DATA_BLOCK "IMAC_STANDBY_RECORD"
TITLE = STANDBY_RECORD
AUTHOR : HottendU
FAMILY : IMAC
VERSION : 0.2


  STRUCT
   STANDBY_No001 : STRUCT
    System : WORD ;
    CmdOS : WORD ;
    MirrorCmdOS : WORD ;
    Test : WORD ;
    AlarmOS : WORD ;
    StatusOS : WORD ;
    SysStatusOS : WORD ;
    Status1 : WORD ;
    Status2 : WORD ;
    Status3 : BYTE ;
    InputEdges : BYTE ;
    AutoEdges : WORD ;
    DataTimeCODelay : STRUCT
     StartTime : DINT ;
     StartEdge : BOOL ;
    END_STRUCT ;
    DataTimeStartingA : STRUCT
     StartTime : DINT ;
     StartEdge : BOOL ;
    END_STRUCT ;
    DataTimeStartingB : STRUCT
     StartTime : DINT ;
     StartEdge : BOOL ;
    END_STRUCT ;
    DataTimeFaultA : STRUCT
     StartTime : DINT ;
     StartEdge : BOOL ;
    END_STRUCT ;
    DataTimeFaultB : STRUCT
     StartTime : DINT ;
     StartEdge : BOOL ;
    END_STRUCT ;
    PCONF : STRUCT 	//// PCONF STANDBY - Instance 001
     Modeswitches : STRUCT
      M0_Spare : BOOL ;	// Spare
      M1_Spare : BOOL ;	// Spare
      M2_Spare : BOOL ;	// Spare
      M3_Spare : BOOL ;	// Spare
      M4_Spare : BOOL ;	// Spare
      M5_Spare : BOOL ;	// Spare
      M6_Spare : BOOL ;	// Spare
      M7_Spare : BOOL ;	// Spare
      M8_Spare : BOOL ;	// Spare
      M9_Spare : BOOL ;	// Spare
      M10_Spare : BOOL ;	// Spare
      M11_Spare : BOOL ;	// Spare
      M12_Spare : BOOL ;	// Spare
      M13_Spare : BOOL ;	// Spare
      M14_Spare : BOOL ;	// Spare
      M15_Test : BOOL ;	// Testbit (1)
     END_STRUCT ;
     DlyTCODelay : TIME  := T#10S;	// Setpoint Action Fault delay
     DlyTStartingA : TIME  := T#3S;	// Setpoint Waiting Delay Slow->Fast
     DlyTStartingB : TIME  := T#3S;	// Setpoint Waiting Delay Fast->Slow
     DlyTFaultA : TIME  := T#2S;	// Setpoint feedback fault delay
     DlyTFaultB : TIME  := T#2S;	// Setpoint change direction
    END_STRUCT ;
   END_STRUCT ;
   STANDBY_No002 : STRUCT
    System : WORD ;
    CmdOS : WORD ;
    MirrorCmdOS : WORD ;
    Test : WORD ;
    AlarmOS : WORD ;
    StatusOS : WORD ;
    SysStatusOS : WORD ;
    Status1 : WORD ;
    Status2 : WORD ;
    Status3 : BYTE ;
    InputEdges : BYTE ;
    AutoEdges : WORD ;
    DataTimeCODelay : STRUCT
     StartTime : DINT ;
     StartEdge : BOOL ;
    END_STRUCT ;
    DataTimeStartingA : STRUCT
     StartTime : DINT ;
     StartEdge : BOOL ;
    END_STRUCT ;
    DataTimeStartingB : STRUCT
     StartTime : DINT ;
     StartEdge : BOOL ;
    END_STRUCT ;
    DataTimeFaultA : STRUCT
     StartTime : DINT ;
     StartEdge : BOOL ;
    END_STRUCT ;
    DataTimeFaultB : STRUCT
     StartTime : DINT ;
     StartEdge : BOOL ;
    END_STRUCT ;
    PCONF : STRUCT 	//// PCONF STANDBY - Instance 002
     Modeswitches : STRUCT
      M0_Spare : BOOL ;	// Spare
      M1_Spare : BOOL ;	// Spare
      M2_Spare : BOOL ;	// Spare
      M3_Spare : BOOL ;	// Spare
      M4_Spare : BOOL ;	// Spare
      M5_Spare : BOOL ;	// Spare
      M6_Spare : BOOL ;	// Spare
      M7_Spare : BOOL ;	// Spare
      M8_Spare : BOOL ;	// Spare
      M9_Spare : BOOL ;	// Spare
      M10_Spare : BOOL ;	// Spare
      M11_Spare : BOOL ;	// Spare
      M12_Spare : BOOL ;	// Spare
      M13_Spare : BOOL ;	// Spare
      M14_Spare : BOOL ;	// Spare
      M15_Test : BOOL ;	// Testbit (1)
     END_STRUCT ;
     DlyTCODelay : TIME ;	// Setpoint Action Fault delay
     DlyTStartingA : TIME ;	// Setpoint Waiting Delay Slow->Fast
     DlyTStartingB : TIME ;	// Setpoint Waiting Delay Fast->Slow
     DlyTFaultA : TIME ;	// Setpoint feedback fault delay
     DlyTFaultB : TIME ;	// Setpoint change direction
    END_STRUCT ;
   END_STRUCT ;
   STANDBY_No003 : STRUCT
    System : WORD ;
    CmdOS : WORD ;
    MirrorCmdOS : WORD ;
    Test : WORD ;
    AlarmOS : WORD ;
    StatusOS : WORD ;
    SysStatusOS : WORD ;
    Status1 : WORD ;
    Status2 : WORD ;
    Status3 : BYTE ;
    InputEdges : BYTE ;
    AutoEdges : WORD ;
    DataTimeCODelay : STRUCT
     StartTime : DINT ;
     StartEdge : BOOL ;
    END_STRUCT ;
    DataTimeStartingA : STRUCT
     StartTime : DINT ;
     StartEdge : BOOL ;
    END_STRUCT ;
    DataTimeStartingB : STRUCT
     StartTime : DINT ;
     StartEdge : BOOL ;
    END_STRUCT ;
    DataTimeFaultA : STRUCT
     StartTime : DINT ;
     StartEdge : BOOL ;
    END_STRUCT ;
    DataTimeFaultB : STRUCT
     StartTime : DINT ;
     StartEdge : BOOL ;
    END_STRUCT ;
    PCONF : STRUCT 	//// PCONF STANDBY - Instance 003
     Modeswitches : STRUCT
      M0_Spare : BOOL ;	// Spare
      M1_Spare : BOOL ;	// Spare
      M2_Spare : BOOL ;	// Spare
      M3_Spare : BOOL ;	// Spare
      M4_Spare : BOOL ;	// Spare
      M5_Spare : BOOL ;	// Spare
      M6_Spare : BOOL ;	// Spare
      M7_Spare : BOOL ;	// Spare
      M8_Spare : BOOL ;	// Spare
      M9_Spare : BOOL ;	// Spare
      M10_Spare : BOOL ;	// Spare
      M11_Spare : BOOL ;	// Spare
      M12_Spare : BOOL ;	// Spare
      M13_Spare : BOOL ;	// Spare
      M14_Spare : BOOL ;	// Spare
      M15_Test : BOOL ;	// Testbit (1)
     END_STRUCT ;
     DlyTCODelay : TIME ;	// Setpoint Action Fault delay
     DlyTStartingA : TIME ;	// Setpoint Waiting Delay Slow->Fast
     DlyTStartingB : TIME ;	// Setpoint Waiting Delay Fast->Slow
     DlyTFaultA : TIME ;	// Setpoint feedback fault delay
     DlyTFaultB : TIME ;	// Setpoint change direction
    END_STRUCT ;
   END_STRUCT ;
   STANDBY_No004 : STRUCT
    System : WORD ;
    CmdOS : WORD ;
    MirrorCmdOS : WORD ;
    Test : WORD ;
    AlarmOS : WORD ;
    StatusOS : WORD ;
    SysStatusOS : WORD ;
    Status1 : WORD ;
    Status2 : WORD ;
    Status3 : BYTE ;
    InputEdges : BYTE ;
    AutoEdges : WORD ;
    DataTimeCODelay : STRUCT
     StartTime : DINT ;
     StartEdge : BOOL ;
    END_STRUCT ;
    DataTimeStartingA : STRUCT
     StartTime : DINT ;
     StartEdge : BOOL ;
    END_STRUCT ;
    DataTimeStartingB : STRUCT
     StartTime : DINT ;
     StartEdge : BOOL ;
    END_STRUCT ;
    DataTimeFaultA : STRUCT
     StartTime : DINT ;
     StartEdge : BOOL ;
    END_STRUCT ;
    DataTimeFaultB : STRUCT
     StartTime : DINT ;
     StartEdge : BOOL ;
    END_STRUCT ;
    PCONF : STRUCT 	//// PCONF STANDBY - Instance 004
     Modeswitches : STRUCT
      M0_Spare : BOOL ;	// Spare
      M1_Spare : BOOL ;	// Spare
      M2_Spare : BOOL ;	// Spare
      M3_Spare : BOOL ;	// Spare
      M4_Spare : BOOL ;	// Spare
      M5_Spare : BOOL ;	// Spare
      M6_Spare : BOOL ;	// Spare
      M7_Spare : BOOL ;	// Spare
      M8_Spare : BOOL ;	// Spare
      M9_Spare : BOOL ;	// Spare
      M10_Spare : BOOL ;	// Spare
      M11_Spare : BOOL ;	// Spare
      M12_Spare : BOOL ;	// Spare
      M13_Spare : BOOL ;	// Spare
      M14_Spare : BOOL ;	// Spare
      M15_Test : BOOL ;	// Testbit (1)
     END_STRUCT ;
     DlyTCODelay : TIME ;	// Setpoint Action Fault delay
     DlyTStartingA : TIME ;	// Setpoint Waiting Delay Slow->Fast
     DlyTStartingB : TIME ;	// Setpoint Waiting Delay Fast->Slow
     DlyTFaultA : TIME ;	// Setpoint feedback fault delay
     DlyTFaultB : TIME ;	// Setpoint change direction
    END_STRUCT ;
   END_STRUCT ;
   STANDBY_No005 : STRUCT
    System : WORD ;
    CmdOS : WORD ;
    MirrorCmdOS : WORD ;
    Test : WORD ;
    AlarmOS : WORD ;
    StatusOS : WORD ;
    SysStatusOS : WORD ;
    Status1 : WORD ;
    Status2 : WORD ;
    Status3 : BYTE ;
    InputEdges : BYTE ;
    AutoEdges : WORD ;
    DataTimeCODelay : STRUCT
     StartTime : DINT ;
     StartEdge : BOOL ;
    END_STRUCT ;
    DataTimeStartingA : STRUCT
     StartTime : DINT ;
     StartEdge : BOOL ;
    END_STRUCT ;
    DataTimeStartingB : STRUCT
     StartTime : DINT ;
     StartEdge : BOOL ;
    END_STRUCT ;
    DataTimeFaultA : STRUCT
     StartTime : DINT ;
     StartEdge : BOOL ;
    END_STRUCT ;
    DataTimeFaultB : STRUCT
     StartTime : DINT ;
     StartEdge : BOOL ;
    END_STRUCT ;
    PCONF : STRUCT 	//// PCONF STANDBY - Instance 005
     Modeswitches : STRUCT
      M0_Spare : BOOL ;	// Spare
      M1_Spare : BOOL ;	// Spare
      M2_Spare : BOOL ;	// Spare
      M3_Spare : BOOL ;	// Spare
      M4_Spare : BOOL ;	// Spare
      M5_Spare : BOOL ;	// Spare
      M6_Spare : BOOL ;	// Spare
      M7_Spare : BOOL ;	// Spare
      M8_Spare : BOOL ;	// Spare
      M9_Spare : BOOL ;	// Spare
      M10_Spare : BOOL ;	// Spare
      M11_Spare : BOOL ;	// Spare
      M12_Spare : BOOL ;	// Spare
      M13_Spare : BOOL ;	// Spare
      M14_Spare : BOOL ;	// Spare
      M15_Test : BOOL ;	// Testbit (1)
     END_STRUCT ;
     DlyTCODelay : TIME ;	// Setpoint Action Fault delay
     DlyTStartingA : TIME ;	// Setpoint Waiting Delay Slow->Fast
     DlyTStartingB : TIME ;	// Setpoint Waiting Delay Fast->Slow
     DlyTFaultA : TIME ;	// Setpoint feedback fault delay
     DlyTFaultB : TIME ;	// Setpoint change direction
    END_STRUCT ;
   END_STRUCT ;
   STANDBY_No006 : STRUCT
    System : WORD ;
    CmdOS : WORD ;
    MirrorCmdOS : WORD ;
    Test : WORD ;
    AlarmOS : WORD ;
    StatusOS : WORD ;
    SysStatusOS : WORD ;
    Status1 : WORD ;
    Status2 : WORD ;
    Status3 : BYTE ;
    InputEdges : BYTE ;
    AutoEdges : WORD ;
    DataTimeCODelay : STRUCT
     StartTime : DINT ;
     StartEdge : BOOL ;
    END_STRUCT ;
    DataTimeStartingA : STRUCT
     StartTime : DINT ;
     StartEdge : BOOL ;
    END_STRUCT ;
    DataTimeStartingB : STRUCT
     StartTime : DINT ;
     StartEdge : BOOL ;
    END_STRUCT ;
    DataTimeFaultA : STRUCT
     StartTime : DINT ;
     StartEdge : BOOL ;
    END_STRUCT ;
    DataTimeFaultB : STRUCT
     StartTime : DINT ;
     StartEdge : BOOL ;
    END_STRUCT ;
    PCONF : STRUCT 	//// PCONF STANDBY - Instance 006
     Modeswitches : STRUCT
      M0_Spare : BOOL ;	// Spare
      M1_Spare : BOOL ;	// Spare
      M2_Spare : BOOL ;	// Spare
      M3_Spare : BOOL ;	// Spare
      M4_Spare : BOOL ;	// Spare
      M5_Spare : BOOL ;	// Spare
      M6_Spare : BOOL ;	// Spare
      M7_Spare : BOOL ;	// Spare
      M8_Spare : BOOL ;	// Spare
      M9_Spare : BOOL ;	// Spare
      M10_Spare : BOOL ;	// Spare
      M11_Spare : BOOL ;	// Spare
      M12_Spare : BOOL ;	// Spare
      M13_Spare : BOOL ;	// Spare
      M14_Spare : BOOL ;	// Spare
      M15_Test : BOOL ;	// Testbit (1)
     END_STRUCT ;
     DlyTCODelay : TIME ;	// Setpoint Action Fault delay
     DlyTStartingA : TIME ;	// Setpoint Waiting Delay Slow->Fast
     DlyTStartingB : TIME ;	// Setpoint Waiting Delay Fast->Slow
     DlyTFaultA : TIME ;	// Setpoint feedback fault delay
     DlyTFaultB : TIME ;	// Setpoint change direction
    END_STRUCT ;
   END_STRUCT ;
   STANDBY_No007 : STRUCT
    System : WORD ;
    CmdOS : WORD ;
    MirrorCmdOS : WORD ;
    Test : WORD ;
    AlarmOS : WORD ;
    StatusOS : WORD ;
    SysStatusOS : WORD ;
    Status1 : WORD ;
    Status2 : WORD ;
    Status3 : BYTE ;
    InputEdges : BYTE ;
    AutoEdges : WORD ;
    DataTimeCODelay : STRUCT
     StartTime : DINT ;
     StartEdge : BOOL ;
    END_STRUCT ;
    DataTimeStartingA : STRUCT
     StartTime : DINT ;
     StartEdge : BOOL ;
    END_STRUCT ;
    DataTimeStartingB : STRUCT
     StartTime : DINT ;
     StartEdge : BOOL ;
    END_STRUCT ;
    DataTimeFaultA : STRUCT
     StartTime : DINT ;
     StartEdge : BOOL ;
    END_STRUCT ;
    DataTimeFaultB : STRUCT
     StartTime : DINT ;
     StartEdge : BOOL ;
    END_STRUCT ;
    PCONF : STRUCT 	//// PCONF STANDBY - Instance 007
     Modeswitches : STRUCT
      M0_Spare : BOOL ;	// Spare
      M1_Spare : BOOL ;	// Spare
      M2_Spare : BOOL ;	// Spare
      M3_Spare : BOOL ;	// Spare
      M4_Spare : BOOL ;	// Spare
      M5_Spare : BOOL ;	// Spare
      M6_Spare : BOOL ;	// Spare
      M7_Spare : BOOL ;	// Spare
      M8_Spare : BOOL ;	// Spare
      M9_Spare : BOOL ;	// Spare
      M10_Spare : BOOL ;	// Spare
      M11_Spare : BOOL ;	// Spare
      M12_Spare : BOOL ;	// Spare
      M13_Spare : BOOL ;	// Spare
      M14_Spare : BOOL ;	// Spare
      M15_Test : BOOL ;	// Testbit (1)
     END_STRUCT ;
     DlyTCODelay : TIME ;	// Setpoint Action Fault delay
     DlyTStartingA : TIME ;	// Setpoint Waiting Delay Slow->Fast
     DlyTStartingB : TIME ;	// Setpoint Waiting Delay Fast->Slow
     DlyTFaultA : TIME ;	// Setpoint feedback fault delay
     DlyTFaultB : TIME ;	// Setpoint change direction
    END_STRUCT ;
   END_STRUCT ;
   STANDBY_No008 : STRUCT
    System : WORD ;
    CmdOS : WORD ;
    MirrorCmdOS : WORD ;
    Test : WORD ;
    AlarmOS : WORD ;
    StatusOS : WORD ;
    SysStatusOS : WORD ;
    Status1 : WORD ;
    Status2 : WORD ;
    Status3 : BYTE ;
    InputEdges : BYTE ;
    AutoEdges : WORD ;
    DataTimeCODelay : STRUCT
     StartTime : DINT ;
     StartEdge : BOOL ;
    END_STRUCT ;
    DataTimeStartingA : STRUCT
     StartTime : DINT ;
     StartEdge : BOOL ;
    END_STRUCT ;
    DataTimeStartingB : STRUCT
     StartTime : DINT ;
     StartEdge : BOOL ;
    END_STRUCT ;
    DataTimeFaultA : STRUCT
     StartTime : DINT ;
     StartEdge : BOOL ;
    END_STRUCT ;
    DataTimeFaultB : STRUCT
     StartTime : DINT ;
     StartEdge : BOOL ;
    END_STRUCT ;
    PCONF : STRUCT 	//// PCONF STANDBY - Instance 008
     Modeswitches : STRUCT
      M0_Spare : BOOL ;	// Spare
      M1_Spare : BOOL ;	// Spare
      M2_Spare : BOOL ;	// Spare
      M3_Spare : BOOL ;	// Spare
      M4_Spare : BOOL ;	// Spare
      M5_Spare : BOOL ;	// Spare
      M6_Spare : BOOL ;	// Spare
      M7_Spare : BOOL ;	// Spare
      M8_Spare : BOOL ;	// Spare
      M9_Spare : BOOL ;	// Spare
      M10_Spare : BOOL ;	// Spare
      M11_Spare : BOOL ;	// Spare
      M12_Spare : BOOL ;	// Spare
      M13_Spare : BOOL ;	// Spare
      M14_Spare : BOOL ;	// Spare
      M15_Test : BOOL ;	// Testbit (1)
     END_STRUCT ;
     DlyTCODelay : TIME ;	// Setpoint Action Fault delay
     DlyTStartingA : TIME ;	// Setpoint Waiting Delay Slow->Fast
     DlyTStartingB : TIME ;	// Setpoint Waiting Delay Fast->Slow
     DlyTFaultA : TIME ;	// Setpoint feedback fault delay
     DlyTFaultB : TIME ;	// Setpoint change direction
    END_STRUCT ;
   END_STRUCT ;
   STANDBY_No009 : STRUCT
    System : WORD ;
    CmdOS : WORD ;
    MirrorCmdOS : WORD ;
    Test : WORD ;
    AlarmOS : WORD ;
    StatusOS : WORD ;
    SysStatusOS : WORD ;
    Status1 : WORD ;
    Status2 : WORD ;
    Status3 : BYTE ;
    InputEdges : BYTE ;
    AutoEdges : WORD ;
    DataTimeCODelay : STRUCT
     StartTime : DINT ;
     StartEdge : BOOL ;
    END_STRUCT ;
    DataTimeStartingA : STRUCT
     StartTime : DINT ;
     StartEdge : BOOL ;
    END_STRUCT ;
    DataTimeStartingB : STRUCT
     StartTime : DINT ;
     StartEdge : BOOL ;
    END_STRUCT ;
    DataTimeFaultA : STRUCT
     StartTime : DINT ;
     StartEdge : BOOL ;
    END_STRUCT ;
    DataTimeFaultB : STRUCT
     StartTime : DINT ;
     StartEdge : BOOL ;
    END_STRUCT ;
    PCONF : STRUCT 	//// PCONF STANDBY - Instance 009
     Modeswitches : STRUCT
      M0_Spare : BOOL ;	// Spare
      M1_Spare : BOOL ;	// Spare
      M2_Spare : BOOL ;	// Spare
      M3_Spare : BOOL ;	// Spare
      M4_Spare : BOOL ;	// Spare
      M5_Spare : BOOL ;	// Spare
      M6_Spare : BOOL ;	// Spare
      M7_Spare : BOOL ;	// Spare
      M8_Spare : BOOL ;	// Spare
      M9_Spare : BOOL ;	// Spare
      M10_Spare : BOOL ;	// Spare
      M11_Spare : BOOL ;	// Spare
      M12_Spare : BOOL ;	// Spare
      M13_Spare : BOOL ;	// Spare
      M14_Spare : BOOL ;	// Spare
      M15_Test : BOOL ;	// Testbit (1)
     END_STRUCT ;
     DlyTCODelay : TIME ;	// Setpoint Action Fault delay
     DlyTStartingA : TIME ;	// Setpoint Waiting Delay Slow->Fast
     DlyTStartingB : TIME ;	// Setpoint Waiting Delay Fast->Slow
     DlyTFaultA : TIME ;	// Setpoint feedback fault delay
     DlyTFaultB : TIME ;	// Setpoint change direction
    END_STRUCT ;
   END_STRUCT ;
   STANDBY_No010 : STRUCT
    System : WORD ;
    CmdOS : WORD ;
    MirrorCmdOS : WORD ;
    Test : WORD ;
    AlarmOS : WORD ;
    StatusOS : WORD ;
    SysStatusOS : WORD ;
    Status1 : WORD ;
    Status2 : WORD ;
    Status3 : BYTE ;
    InputEdges : BYTE ;
    AutoEdges : WORD ;
    DataTimeCODelay : STRUCT
     StartTime : DINT ;
     StartEdge : BOOL ;
    END_STRUCT ;
    DataTimeStartingA : STRUCT
     StartTime : DINT ;
     StartEdge : BOOL ;
    END_STRUCT ;
    DataTimeStartingB : STRUCT
     StartTime : DINT ;
     StartEdge : BOOL ;
    END_STRUCT ;
    DataTimeFaultA : STRUCT
     StartTime : DINT ;
     StartEdge : BOOL ;
    END_STRUCT ;
    DataTimeFaultB : STRUCT
     StartTime : DINT ;
     StartEdge : BOOL ;
    END_STRUCT ;
    PCONF : STRUCT 	//// PCONF STANDBY - Instance 010
     Modeswitches : STRUCT
      M0_Spare : BOOL ;	// Spare
      M1_Spare : BOOL ;	// Spare
      M2_Spare : BOOL ;	// Spare
      M3_Spare : BOOL ;	// Spare
      M4_Spare : BOOL ;	// Spare
      M5_Spare : BOOL ;	// Spare
      M6_Spare : BOOL ;	// Spare
      M7_Spare : BOOL ;	// Spare
      M8_Spare : BOOL ;	// Spare
      M9_Spare : BOOL ;	// Spare
      M10_Spare : BOOL ;	// Spare
      M11_Spare : BOOL ;	// Spare
      M12_Spare : BOOL ;	// Spare
      M13_Spare : BOOL ;	// Spare
      M14_Spare : BOOL ;	// Spare
      M15_Test : BOOL ;	// Testbit (1)
     END_STRUCT ;
     DlyTCODelay : TIME ;	// Setpoint Action Fault delay
     DlyTStartingA : TIME ;	// Setpoint Waiting Delay Slow->Fast
     DlyTStartingB : TIME ;	// Setpoint Waiting Delay Fast->Slow
     DlyTFaultA : TIME ;	// Setpoint feedback fault delay
     DlyTFaultB : TIME ;	// Setpoint change direction
    END_STRUCT ;
   END_STRUCT ;
  END_STRUCT ;
BEGIN
   STANDBY_No001.System := W#16#0;
   STANDBY_No001.CmdOS := W#16#0;
   STANDBY_No001.MirrorCmdOS := W#16#0;
   STANDBY_No001.Test := W#16#0;
   STANDBY_No001.AlarmOS := W#16#0;
   STANDBY_No001.StatusOS := W#16#0;
   STANDBY_No001.SysStatusOS := W#16#0;
   STANDBY_No001.Status1 := W#16#0;
   STANDBY_No001.Status2 := W#16#0;
   STANDBY_No001.Status3 := B#16#0;
   STANDBY_No001.InputEdges := B#16#0;
   STANDBY_No001.AutoEdges := W#16#0;
   STANDBY_No001.DataTimeCODelay.StartTime := L#0;
   STANDBY_No001.DataTimeCODelay.StartEdge := FALSE;
   STANDBY_No001.DataTimeStartingA.StartTime := L#0;
   STANDBY_No001.DataTimeStartingA.StartEdge := FALSE;
   STANDBY_No001.DataTimeStartingB.StartTime := L#0;
   STANDBY_No001.DataTimeStartingB.StartEdge := FALSE;
   STANDBY_No001.DataTimeFaultA.StartTime := L#0;
   STANDBY_No001.DataTimeFaultA.StartEdge := FALSE;
   STANDBY_No001.DataTimeFaultB.StartTime := L#0;
   STANDBY_No001.DataTimeFaultB.StartEdge := FALSE;
   STANDBY_No001.PCONF.Modeswitches.M0_Spare := FALSE;
   STANDBY_No001.PCONF.Modeswitches.M1_Spare := FALSE;
   STANDBY_No001.PCONF.Modeswitches.M2_Spare := FALSE;
   STANDBY_No001.PCONF.Modeswitches.M3_Spare := FALSE;
   STANDBY_No001.PCONF.Modeswitches.M4_Spare := FALSE;
   STANDBY_No001.PCONF.Modeswitches.M5_Spare := FALSE;
   STANDBY_No001.PCONF.Modeswitches.M6_Spare := FALSE;
   STANDBY_No001.PCONF.Modeswitches.M7_Spare := FALSE;
   STANDBY_No001.PCONF.Modeswitches.M8_Spare := FALSE;
   STANDBY_No001.PCONF.Modeswitches.M9_Spare := FALSE;
   STANDBY_No001.PCONF.Modeswitches.M10_Spare := FALSE;
   STANDBY_No001.PCONF.Modeswitches.M11_Spare := FALSE;
   STANDBY_No001.PCONF.Modeswitches.M12_Spare := FALSE;
   STANDBY_No001.PCONF.Modeswitches.M13_Spare := FALSE;
   STANDBY_No001.PCONF.Modeswitches.M14_Spare := FALSE;
   STANDBY_No001.PCONF.Modeswitches.M15_Test := FALSE;
   STANDBY_No001.PCONF.DlyTCODelay := T#10S;
   STANDBY_No001.PCONF.DlyTStartingA := T#3S;
   STANDBY_No001.PCONF.DlyTStartingB := T#3S;
   STANDBY_No001.PCONF.DlyTFaultA := T#2S;
   STANDBY_No001.PCONF.DlyTFaultB := T#2S;
   STANDBY_No002.System := W#16#0;
   STANDBY_No002.CmdOS := W#16#0;
   STANDBY_No002.MirrorCmdOS := W#16#0;
   STANDBY_No002.Test := W#16#0;
   STANDBY_No002.AlarmOS := W#16#0;
   STANDBY_No002.StatusOS := W#16#0;
   STANDBY_No002.SysStatusOS := W#16#0;
   STANDBY_No002.Status1 := W#16#0;
   STANDBY_No002.Status2 := W#16#0;
   STANDBY_No002.Status3 := B#16#0;
   STANDBY_No002.InputEdges := B#16#0;
   STANDBY_No002.AutoEdges := W#16#0;
   STANDBY_No002.DataTimeCODelay.StartTime := L#0;
   STANDBY_No002.DataTimeCODelay.StartEdge := FALSE;
   STANDBY_No002.DataTimeStartingA.StartTime := L#0;
   STANDBY_No002.DataTimeStartingA.StartEdge := FALSE;
   STANDBY_No002.DataTimeStartingB.StartTime := L#0;
   STANDBY_No002.DataTimeStartingB.StartEdge := FALSE;
   STANDBY_No002.DataTimeFaultA.StartTime := L#0;
   STANDBY_No002.DataTimeFaultA.StartEdge := FALSE;
   STANDBY_No002.DataTimeFaultB.StartTime := L#0;
   STANDBY_No002.DataTimeFaultB.StartEdge := FALSE;
   STANDBY_No002.PCONF.Modeswitches.M0_Spare := FALSE;
   STANDBY_No002.PCONF.Modeswitches.M1_Spare := FALSE;
   STANDBY_No002.PCONF.Modeswitches.M2_Spare := FALSE;
   STANDBY_No002.PCONF.Modeswitches.M3_Spare := FALSE;
   STANDBY_No002.PCONF.Modeswitches.M4_Spare := FALSE;
   STANDBY_No002.PCONF.Modeswitches.M5_Spare := FALSE;
   STANDBY_No002.PCONF.Modeswitches.M6_Spare := FALSE;
   STANDBY_No002.PCONF.Modeswitches.M7_Spare := FALSE;
   STANDBY_No002.PCONF.Modeswitches.M8_Spare := FALSE;
   STANDBY_No002.PCONF.Modeswitches.M9_Spare := FALSE;
   STANDBY_No002.PCONF.Modeswitches.M10_Spare := FALSE;
   STANDBY_No002.PCONF.Modeswitches.M11_Spare := FALSE;
   STANDBY_No002.PCONF.Modeswitches.M12_Spare := FALSE;
   STANDBY_No002.PCONF.Modeswitches.M13_Spare := FALSE;
   STANDBY_No002.PCONF.Modeswitches.M14_Spare := FALSE;
   STANDBY_No002.PCONF.Modeswitches.M15_Test := FALSE;
   STANDBY_No002.PCONF.DlyTCODelay := T#0MS;
   STANDBY_No002.PCONF.DlyTStartingA := T#0MS;
   STANDBY_No002.PCONF.DlyTStartingB := T#0MS;
   STANDBY_No002.PCONF.DlyTFaultA := T#0MS;
   STANDBY_No002.PCONF.DlyTFaultB := T#0MS;
   STANDBY_No003.System := W#16#0;
   STANDBY_No003.CmdOS := W#16#0;
   STANDBY_No003.MirrorCmdOS := W#16#0;
   STANDBY_No003.Test := W#16#0;
   STANDBY_No003.AlarmOS := W#16#0;
   STANDBY_No003.StatusOS := W#16#0;
   STANDBY_No003.SysStatusOS := W#16#0;
   STANDBY_No003.Status1 := W#16#0;
   STANDBY_No003.Status2 := W#16#0;
   STANDBY_No003.Status3 := B#16#0;
   STANDBY_No003.InputEdges := B#16#0;
   STANDBY_No003.AutoEdges := W#16#0;
   STANDBY_No003.DataTimeCODelay.StartTime := L#0;
   STANDBY_No003.DataTimeCODelay.StartEdge := FALSE;
   STANDBY_No003.DataTimeStartingA.StartTime := L#0;
   STANDBY_No003.DataTimeStartingA.StartEdge := FALSE;
   STANDBY_No003.DataTimeStartingB.StartTime := L#0;
   STANDBY_No003.DataTimeStartingB.StartEdge := FALSE;
   STANDBY_No003.DataTimeFaultA.StartTime := L#0;
   STANDBY_No003.DataTimeFaultA.StartEdge := FALSE;
   STANDBY_No003.DataTimeFaultB.StartTime := L#0;
   STANDBY_No003.DataTimeFaultB.StartEdge := FALSE;
   STANDBY_No003.PCONF.Modeswitches.M0_Spare := FALSE;
   STANDBY_No003.PCONF.Modeswitches.M1_Spare := FALSE;
   STANDBY_No003.PCONF.Modeswitches.M2_Spare := FALSE;
   STANDBY_No003.PCONF.Modeswitches.M3_Spare := FALSE;
   STANDBY_No003.PCONF.Modeswitches.M4_Spare := FALSE;
   STANDBY_No003.PCONF.Modeswitches.M5_Spare := FALSE;
   STANDBY_No003.PCONF.Modeswitches.M6_Spare := FALSE;
   STANDBY_No003.PCONF.Modeswitches.M7_Spare := FALSE;
   STANDBY_No003.PCONF.Modeswitches.M8_Spare := FALSE;
   STANDBY_No003.PCONF.Modeswitches.M9_Spare := FALSE;
   STANDBY_No003.PCONF.Modeswitches.M10_Spare := FALSE;
   STANDBY_No003.PCONF.Modeswitches.M11_Spare := FALSE;
   STANDBY_No003.PCONF.Modeswitches.M12_Spare := FALSE;
   STANDBY_No003.PCONF.Modeswitches.M13_Spare := FALSE;
   STANDBY_No003.PCONF.Modeswitches.M14_Spare := FALSE;
   STANDBY_No003.PCONF.Modeswitches.M15_Test := FALSE;
   STANDBY_No003.PCONF.DlyTCODelay := T#0MS;
   STANDBY_No003.PCONF.DlyTStartingA := T#0MS;
   STANDBY_No003.PCONF.DlyTStartingB := T#0MS;
   STANDBY_No003.PCONF.DlyTFaultA := T#0MS;
   STANDBY_No003.PCONF.DlyTFaultB := T#0MS;
   STANDBY_No004.System := W#16#0;
   STANDBY_No004.CmdOS := W#16#0;
   STANDBY_No004.MirrorCmdOS := W#16#0;
   STANDBY_No004.Test := W#16#0;
   STANDBY_No004.AlarmOS := W#16#0;
   STANDBY_No004.StatusOS := W#16#0;
   STANDBY_No004.SysStatusOS := W#16#0;
   STANDBY_No004.Status1 := W#16#0;
   STANDBY_No004.Status2 := W#16#0;
   STANDBY_No004.Status3 := B#16#0;
   STANDBY_No004.InputEdges := B#16#0;
   STANDBY_No004.AutoEdges := W#16#0;
   STANDBY_No004.DataTimeCODelay.StartTime := L#0;
   STANDBY_No004.DataTimeCODelay.StartEdge := FALSE;
   STANDBY_No004.DataTimeStartingA.StartTime := L#0;
   STANDBY_No004.DataTimeStartingA.StartEdge := FALSE;
   STANDBY_No004.DataTimeStartingB.StartTime := L#0;
   STANDBY_No004.DataTimeStartingB.StartEdge := FALSE;
   STANDBY_No004.DataTimeFaultA.StartTime := L#0;
   STANDBY_No004.DataTimeFaultA.StartEdge := FALSE;
   STANDBY_No004.DataTimeFaultB.StartTime := L#0;
   STANDBY_No004.DataTimeFaultB.StartEdge := FALSE;
   STANDBY_No004.PCONF.Modeswitches.M0_Spare := FALSE;
   STANDBY_No004.PCONF.Modeswitches.M1_Spare := FALSE;
   STANDBY_No004.PCONF.Modeswitches.M2_Spare := FALSE;
   STANDBY_No004.PCONF.Modeswitches.M3_Spare := FALSE;
   STANDBY_No004.PCONF.Modeswitches.M4_Spare := FALSE;
   STANDBY_No004.PCONF.Modeswitches.M5_Spare := FALSE;
   STANDBY_No004.PCONF.Modeswitches.M6_Spare := FALSE;
   STANDBY_No004.PCONF.Modeswitches.M7_Spare := FALSE;
   STANDBY_No004.PCONF.Modeswitches.M8_Spare := FALSE;
   STANDBY_No004.PCONF.Modeswitches.M9_Spare := FALSE;
   STANDBY_No004.PCONF.Modeswitches.M10_Spare := FALSE;
   STANDBY_No004.PCONF.Modeswitches.M11_Spare := FALSE;
   STANDBY_No004.PCONF.Modeswitches.M12_Spare := FALSE;
   STANDBY_No004.PCONF.Modeswitches.M13_Spare := FALSE;
   STANDBY_No004.PCONF.Modeswitches.M14_Spare := FALSE;
   STANDBY_No004.PCONF.Modeswitches.M15_Test := FALSE;
   STANDBY_No004.PCONF.DlyTCODelay := T#0MS;
   STANDBY_No004.PCONF.DlyTStartingA := T#0MS;
   STANDBY_No004.PCONF.DlyTStartingB := T#0MS;
   STANDBY_No004.PCONF.DlyTFaultA := T#0MS;
   STANDBY_No004.PCONF.DlyTFaultB := T#0MS;
   STANDBY_No005.System := W#16#0;
   STANDBY_No005.CmdOS := W#16#0;
   STANDBY_No005.MirrorCmdOS := W#16#0;
   STANDBY_No005.Test := W#16#0;
   STANDBY_No005.AlarmOS := W#16#0;
   STANDBY_No005.StatusOS := W#16#0;
   STANDBY_No005.SysStatusOS := W#16#0;
   STANDBY_No005.Status1 := W#16#0;
   STANDBY_No005.Status2 := W#16#0;
   STANDBY_No005.Status3 := B#16#0;
   STANDBY_No005.InputEdges := B#16#0;
   STANDBY_No005.AutoEdges := W#16#0;
   STANDBY_No005.DataTimeCODelay.StartTime := L#0;
   STANDBY_No005.DataTimeCODelay.StartEdge := FALSE;
   STANDBY_No005.DataTimeStartingA.StartTime := L#0;
   STANDBY_No005.DataTimeStartingA.StartEdge := FALSE;
   STANDBY_No005.DataTimeStartingB.StartTime := L#0;
   STANDBY_No005.DataTimeStartingB.StartEdge := FALSE;
   STANDBY_No005.DataTimeFaultA.StartTime := L#0;
   STANDBY_No005.DataTimeFaultA.StartEdge := FALSE;
   STANDBY_No005.DataTimeFaultB.StartTime := L#0;
   STANDBY_No005.DataTimeFaultB.StartEdge := FALSE;
   STANDBY_No005.PCONF.Modeswitches.M0_Spare := FALSE;
   STANDBY_No005.PCONF.Modeswitches.M1_Spare := FALSE;
   STANDBY_No005.PCONF.Modeswitches.M2_Spare := FALSE;
   STANDBY_No005.PCONF.Modeswitches.M3_Spare := FALSE;
   STANDBY_No005.PCONF.Modeswitches.M4_Spare := FALSE;
   STANDBY_No005.PCONF.Modeswitches.M5_Spare := FALSE;
   STANDBY_No005.PCONF.Modeswitches.M6_Spare := FALSE;
   STANDBY_No005.PCONF.Modeswitches.M7_Spare := FALSE;
   STANDBY_No005.PCONF.Modeswitches.M8_Spare := FALSE;
   STANDBY_No005.PCONF.Modeswitches.M9_Spare := FALSE;
   STANDBY_No005.PCONF.Modeswitches.M10_Spare := FALSE;
   STANDBY_No005.PCONF.Modeswitches.M11_Spare := FALSE;
   STANDBY_No005.PCONF.Modeswitches.M12_Spare := FALSE;
   STANDBY_No005.PCONF.Modeswitches.M13_Spare := FALSE;
   STANDBY_No005.PCONF.Modeswitches.M14_Spare := FALSE;
   STANDBY_No005.PCONF.Modeswitches.M15_Test := FALSE;
   STANDBY_No005.PCONF.DlyTCODelay := T#0MS;
   STANDBY_No005.PCONF.DlyTStartingA := T#0MS;
   STANDBY_No005.PCONF.DlyTStartingB := T#0MS;
   STANDBY_No005.PCONF.DlyTFaultA := T#0MS;
   STANDBY_No005.PCONF.DlyTFaultB := T#0MS;
   STANDBY_No006.System := W#16#0;
   STANDBY_No006.CmdOS := W#16#0;
   STANDBY_No006.MirrorCmdOS := W#16#0;
   STANDBY_No006.Test := W#16#0;
   STANDBY_No006.AlarmOS := W#16#0;
   STANDBY_No006.StatusOS := W#16#0;
   STANDBY_No006.SysStatusOS := W#16#0;
   STANDBY_No006.Status1 := W#16#0;
   STANDBY_No006.Status2 := W#16#0;
   STANDBY_No006.Status3 := B#16#0;
   STANDBY_No006.InputEdges := B#16#0;
   STANDBY_No006.AutoEdges := W#16#0;
   STANDBY_No006.DataTimeCODelay.StartTime := L#0;
   STANDBY_No006.DataTimeCODelay.StartEdge := FALSE;
   STANDBY_No006.DataTimeStartingA.StartTime := L#0;
   STANDBY_No006.DataTimeStartingA.StartEdge := FALSE;
   STANDBY_No006.DataTimeStartingB.StartTime := L#0;
   STANDBY_No006.DataTimeStartingB.StartEdge := FALSE;
   STANDBY_No006.DataTimeFaultA.StartTime := L#0;
   STANDBY_No006.DataTimeFaultA.StartEdge := FALSE;
   STANDBY_No006.DataTimeFaultB.StartTime := L#0;
   STANDBY_No006.DataTimeFaultB.StartEdge := FALSE;
   STANDBY_No006.PCONF.Modeswitches.M0_Spare := FALSE;
   STANDBY_No006.PCONF.Modeswitches.M1_Spare := FALSE;
   STANDBY_No006.PCONF.Modeswitches.M2_Spare := FALSE;
   STANDBY_No006.PCONF.Modeswitches.M3_Spare := FALSE;
   STANDBY_No006.PCONF.Modeswitches.M4_Spare := FALSE;
   STANDBY_No006.PCONF.Modeswitches.M5_Spare := FALSE;
   STANDBY_No006.PCONF.Modeswitches.M6_Spare := FALSE;
   STANDBY_No006.PCONF.Modeswitches.M7_Spare := FALSE;
   STANDBY_No006.PCONF.Modeswitches.M8_Spare := FALSE;
   STANDBY_No006.PCONF.Modeswitches.M9_Spare := FALSE;
   STANDBY_No006.PCONF.Modeswitches.M10_Spare := FALSE;
   STANDBY_No006.PCONF.Modeswitches.M11_Spare := FALSE;
   STANDBY_No006.PCONF.Modeswitches.M12_Spare := FALSE;
   STANDBY_No006.PCONF.Modeswitches.M13_Spare := FALSE;
   STANDBY_No006.PCONF.Modeswitches.M14_Spare := FALSE;
   STANDBY_No006.PCONF.Modeswitches.M15_Test := FALSE;
   STANDBY_No006.PCONF.DlyTCODelay := T#0MS;
   STANDBY_No006.PCONF.DlyTStartingA := T#0MS;
   STANDBY_No006.PCONF.DlyTStartingB := T#0MS;
   STANDBY_No006.PCONF.DlyTFaultA := T#0MS;
   STANDBY_No006.PCONF.DlyTFaultB := T#0MS;
   STANDBY_No007.System := W#16#0;
   STANDBY_No007.CmdOS := W#16#0;
   STANDBY_No007.MirrorCmdOS := W#16#0;
   STANDBY_No007.Test := W#16#0;
   STANDBY_No007.AlarmOS := W#16#0;
   STANDBY_No007.StatusOS := W#16#0;
   STANDBY_No007.SysStatusOS := W#16#0;
   STANDBY_No007.Status1 := W#16#0;
   STANDBY_No007.Status2 := W#16#0;
   STANDBY_No007.Status3 := B#16#0;
   STANDBY_No007.InputEdges := B#16#0;
   STANDBY_No007.AutoEdges := W#16#0;
   STANDBY_No007.DataTimeCODelay.StartTime := L#0;
   STANDBY_No007.DataTimeCODelay.StartEdge := FALSE;
   STANDBY_No007.DataTimeStartingA.StartTime := L#0;
   STANDBY_No007.DataTimeStartingA.StartEdge := FALSE;
   STANDBY_No007.DataTimeStartingB.StartTime := L#0;
   STANDBY_No007.DataTimeStartingB.StartEdge := FALSE;
   STANDBY_No007.DataTimeFaultA.StartTime := L#0;
   STANDBY_No007.DataTimeFaultA.StartEdge := FALSE;
   STANDBY_No007.DataTimeFaultB.StartTime := L#0;
   STANDBY_No007.DataTimeFaultB.StartEdge := FALSE;
   STANDBY_No007.PCONF.Modeswitches.M0_Spare := FALSE;
   STANDBY_No007.PCONF.Modeswitches.M1_Spare := FALSE;
   STANDBY_No007.PCONF.Modeswitches.M2_Spare := FALSE;
   STANDBY_No007.PCONF.Modeswitches.M3_Spare := FALSE;
   STANDBY_No007.PCONF.Modeswitches.M4_Spare := FALSE;
   STANDBY_No007.PCONF.Modeswitches.M5_Spare := FALSE;
   STANDBY_No007.PCONF.Modeswitches.M6_Spare := FALSE;
   STANDBY_No007.PCONF.Modeswitches.M7_Spare := FALSE;
   STANDBY_No007.PCONF.Modeswitches.M8_Spare := FALSE;
   STANDBY_No007.PCONF.Modeswitches.M9_Spare := FALSE;
   STANDBY_No007.PCONF.Modeswitches.M10_Spare := FALSE;
   STANDBY_No007.PCONF.Modeswitches.M11_Spare := FALSE;
   STANDBY_No007.PCONF.Modeswitches.M12_Spare := FALSE;
   STANDBY_No007.PCONF.Modeswitches.M13_Spare := FALSE;
   STANDBY_No007.PCONF.Modeswitches.M14_Spare := FALSE;
   STANDBY_No007.PCONF.Modeswitches.M15_Test := FALSE;
   STANDBY_No007.PCONF.DlyTCODelay := T#0MS;
   STANDBY_No007.PCONF.DlyTStartingA := T#0MS;
   STANDBY_No007.PCONF.DlyTStartingB := T#0MS;
   STANDBY_No007.PCONF.DlyTFaultA := T#0MS;
   STANDBY_No007.PCONF.DlyTFaultB := T#0MS;
   STANDBY_No008.System := W#16#0;
   STANDBY_No008.CmdOS := W#16#0;
   STANDBY_No008.MirrorCmdOS := W#16#0;
   STANDBY_No008.Test := W#16#0;
   STANDBY_No008.AlarmOS := W#16#0;
   STANDBY_No008.StatusOS := W#16#0;
   STANDBY_No008.SysStatusOS := W#16#0;
   STANDBY_No008.Status1 := W#16#0;
   STANDBY_No008.Status2 := W#16#0;
   STANDBY_No008.Status3 := B#16#0;
   STANDBY_No008.InputEdges := B#16#0;
   STANDBY_No008.AutoEdges := W#16#0;
   STANDBY_No008.DataTimeCODelay.StartTime := L#0;
   STANDBY_No008.DataTimeCODelay.StartEdge := FALSE;
   STANDBY_No008.DataTimeStartingA.StartTime := L#0;
   STANDBY_No008.DataTimeStartingA.StartEdge := FALSE;
   STANDBY_No008.DataTimeStartingB.StartTime := L#0;
   STANDBY_No008.DataTimeStartingB.StartEdge := FALSE;
   STANDBY_No008.DataTimeFaultA.StartTime := L#0;
   STANDBY_No008.DataTimeFaultA.StartEdge := FALSE;
   STANDBY_No008.DataTimeFaultB.StartTime := L#0;
   STANDBY_No008.DataTimeFaultB.StartEdge := FALSE;
   STANDBY_No008.PCONF.Modeswitches.M0_Spare := FALSE;
   STANDBY_No008.PCONF.Modeswitches.M1_Spare := FALSE;
   STANDBY_No008.PCONF.Modeswitches.M2_Spare := FALSE;
   STANDBY_No008.PCONF.Modeswitches.M3_Spare := FALSE;
   STANDBY_No008.PCONF.Modeswitches.M4_Spare := FALSE;
   STANDBY_No008.PCONF.Modeswitches.M5_Spare := FALSE;
   STANDBY_No008.PCONF.Modeswitches.M6_Spare := FALSE;
   STANDBY_No008.PCONF.Modeswitches.M7_Spare := FALSE;
   STANDBY_No008.PCONF.Modeswitches.M8_Spare := FALSE;
   STANDBY_No008.PCONF.Modeswitches.M9_Spare := FALSE;
   STANDBY_No008.PCONF.Modeswitches.M10_Spare := FALSE;
   STANDBY_No008.PCONF.Modeswitches.M11_Spare := FALSE;
   STANDBY_No008.PCONF.Modeswitches.M12_Spare := FALSE;
   STANDBY_No008.PCONF.Modeswitches.M13_Spare := FALSE;
   STANDBY_No008.PCONF.Modeswitches.M14_Spare := FALSE;
   STANDBY_No008.PCONF.Modeswitches.M15_Test := FALSE;
   STANDBY_No008.PCONF.DlyTCODelay := T#0MS;
   STANDBY_No008.PCONF.DlyTStartingA := T#0MS;
   STANDBY_No008.PCONF.DlyTStartingB := T#0MS;
   STANDBY_No008.PCONF.DlyTFaultA := T#0MS;
   STANDBY_No008.PCONF.DlyTFaultB := T#0MS;
   STANDBY_No009.System := W#16#0;
   STANDBY_No009.CmdOS := W#16#0;
   STANDBY_No009.MirrorCmdOS := W#16#0;
   STANDBY_No009.Test := W#16#0;
   STANDBY_No009.AlarmOS := W#16#0;
   STANDBY_No009.StatusOS := W#16#0;
   STANDBY_No009.SysStatusOS := W#16#0;
   STANDBY_No009.Status1 := W#16#0;
   STANDBY_No009.Status2 := W#16#0;
   STANDBY_No009.Status3 := B#16#0;
   STANDBY_No009.InputEdges := B#16#0;
   STANDBY_No009.AutoEdges := W#16#0;
   STANDBY_No009.DataTimeCODelay.StartTime := L#0;
   STANDBY_No009.DataTimeCODelay.StartEdge := FALSE;
   STANDBY_No009.DataTimeStartingA.StartTime := L#0;
   STANDBY_No009.DataTimeStartingA.StartEdge := FALSE;
   STANDBY_No009.DataTimeStartingB.StartTime := L#0;
   STANDBY_No009.DataTimeStartingB.StartEdge := FALSE;
   STANDBY_No009.DataTimeFaultA.StartTime := L#0;
   STANDBY_No009.DataTimeFaultA.StartEdge := FALSE;
   STANDBY_No009.DataTimeFaultB.StartTime := L#0;
   STANDBY_No009.DataTimeFaultB.StartEdge := FALSE;
   STANDBY_No009.PCONF.Modeswitches.M0_Spare := FALSE;
   STANDBY_No009.PCONF.Modeswitches.M1_Spare := FALSE;
   STANDBY_No009.PCONF.Modeswitches.M2_Spare := FALSE;
   STANDBY_No009.PCONF.Modeswitches.M3_Spare := FALSE;
   STANDBY_No009.PCONF.Modeswitches.M4_Spare := FALSE;
   STANDBY_No009.PCONF.Modeswitches.M5_Spare := FALSE;
   STANDBY_No009.PCONF.Modeswitches.M6_Spare := FALSE;
   STANDBY_No009.PCONF.Modeswitches.M7_Spare := FALSE;
   STANDBY_No009.PCONF.Modeswitches.M8_Spare := FALSE;
   STANDBY_No009.PCONF.Modeswitches.M9_Spare := FALSE;
   STANDBY_No009.PCONF.Modeswitches.M10_Spare := FALSE;
   STANDBY_No009.PCONF.Modeswitches.M11_Spare := FALSE;
   STANDBY_No009.PCONF.Modeswitches.M12_Spare := FALSE;
   STANDBY_No009.PCONF.Modeswitches.M13_Spare := FALSE;
   STANDBY_No009.PCONF.Modeswitches.M14_Spare := FALSE;
   STANDBY_No009.PCONF.Modeswitches.M15_Test := FALSE;
   STANDBY_No009.PCONF.DlyTCODelay := T#0MS;
   STANDBY_No009.PCONF.DlyTStartingA := T#0MS;
   STANDBY_No009.PCONF.DlyTStartingB := T#0MS;
   STANDBY_No009.PCONF.DlyTFaultA := T#0MS;
   STANDBY_No009.PCONF.DlyTFaultB := T#0MS;
   STANDBY_No010.System := W#16#0;
   STANDBY_No010.CmdOS := W#16#0;
   STANDBY_No010.MirrorCmdOS := W#16#0;
   STANDBY_No010.Test := W#16#0;
   STANDBY_No010.AlarmOS := W#16#0;
   STANDBY_No010.StatusOS := W#16#0;
   STANDBY_No010.SysStatusOS := W#16#0;
   STANDBY_No010.Status1 := W#16#0;
   STANDBY_No010.Status2 := W#16#0;
   STANDBY_No010.Status3 := B#16#0;
   STANDBY_No010.InputEdges := B#16#0;
   STANDBY_No010.AutoEdges := W#16#0;
   STANDBY_No010.DataTimeCODelay.StartTime := L#0;
   STANDBY_No010.DataTimeCODelay.StartEdge := FALSE;
   STANDBY_No010.DataTimeStartingA.StartTime := L#0;
   STANDBY_No010.DataTimeStartingA.StartEdge := FALSE;
   STANDBY_No010.DataTimeStartingB.StartTime := L#0;
   STANDBY_No010.DataTimeStartingB.StartEdge := FALSE;
   STANDBY_No010.DataTimeFaultA.StartTime := L#0;
   STANDBY_No010.DataTimeFaultA.StartEdge := FALSE;
   STANDBY_No010.DataTimeFaultB.StartTime := L#0;
   STANDBY_No010.DataTimeFaultB.StartEdge := FALSE;
   STANDBY_No010.PCONF.Modeswitches.M0_Spare := FALSE;
   STANDBY_No010.PCONF.Modeswitches.M1_Spare := FALSE;
   STANDBY_No010.PCONF.Modeswitches.M2_Spare := FALSE;
   STANDBY_No010.PCONF.Modeswitches.M3_Spare := FALSE;
   STANDBY_No010.PCONF.Modeswitches.M4_Spare := FALSE;
   STANDBY_No010.PCONF.Modeswitches.M5_Spare := FALSE;
   STANDBY_No010.PCONF.Modeswitches.M6_Spare := FALSE;
   STANDBY_No010.PCONF.Modeswitches.M7_Spare := FALSE;
   STANDBY_No010.PCONF.Modeswitches.M8_Spare := FALSE;
   STANDBY_No010.PCONF.Modeswitches.M9_Spare := FALSE;
   STANDBY_No010.PCONF.Modeswitches.M10_Spare := FALSE;
   STANDBY_No010.PCONF.Modeswitches.M11_Spare := FALSE;
   STANDBY_No010.PCONF.Modeswitches.M12_Spare := FALSE;
   STANDBY_No010.PCONF.Modeswitches.M13_Spare := FALSE;
   STANDBY_No010.PCONF.Modeswitches.M14_Spare := FALSE;
   STANDBY_No010.PCONF.Modeswitches.M15_Test := FALSE;
   STANDBY_No010.PCONF.DlyTCODelay := T#0MS;
   STANDBY_No010.PCONF.DlyTStartingA := T#0MS;
   STANDBY_No010.PCONF.DlyTStartingB := T#0MS;
   STANDBY_No010.PCONF.DlyTFaultA := T#0MS;
   STANDBY_No010.PCONF.DlyTFaultB := T#0MS;
END_DATA_BLOCK

